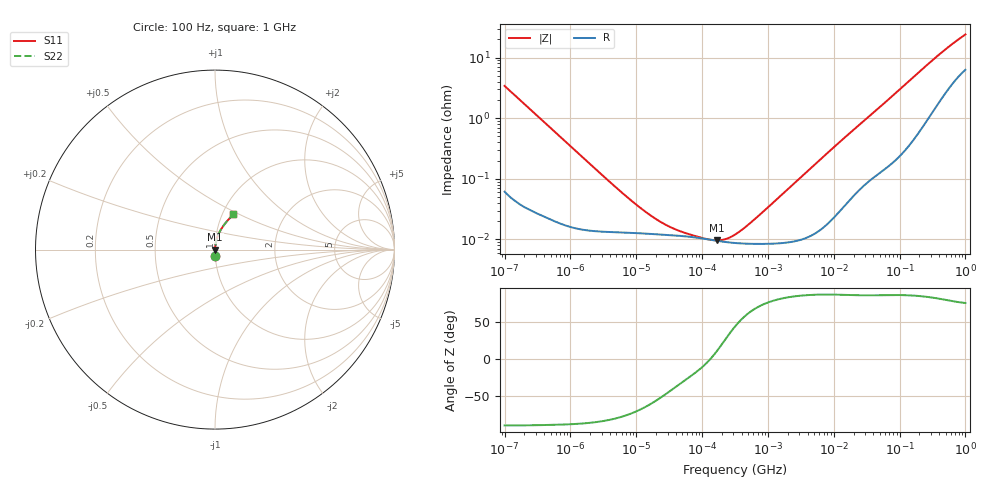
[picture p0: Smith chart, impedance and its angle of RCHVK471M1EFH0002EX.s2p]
! RCHVK471M1EFH0002EX  S-PARAMETER MODEL  (AEC-Q200 qualified)
! Model Generated by ELNA Corporation (http://www.ty-top.com)
! Version 1.0
! ELNA Control No. 240315
! Copyright (c) 2020 ELNA CO.,LTD. All Rights Reserved.
! Products Name : CONDUCTIVE POLYMER HYBRID ALUMINUM ELECTROLYTIC CAPACITORS
! Characteristics :
!  Capacitance  :  470uF  ,  Rated voltage  :  16V
!  Operating Temp. Range  :  -55 to +125 degC  ,  Endurance  :  4000hr at 125 degC
!  Dimension D  :  10mm  ,  Dimension L  :  10mm
! Frequency Range : 100Hz - 1GHz
! External Node Assignments :
!  1  o---| |---o  2
# MHz S RI R 50
!Freq[MHz].  S11 Real  S11 Imag  S21 Real  S21 Imag  S12 Real  S12 Imag  S22 Real  S22 Imag
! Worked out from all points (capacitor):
!   401 points, 100 Hz to 1 GHz, reference 50 ohm
!   read as one part in series: C = 467 uF near 108 Hz
!   lowest |Z| = 9.67 mohm at 166 kHz (marker M1)
!   series resonance near 133.9 kHz, so ESL is about 3 nH
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0.0001  0.00177 -0.034  0.9982 0.034  0.9982 0.034  0.00177 -0.034
0.000113  0.00145 -0.0302  0.9985 0.0302  0.9985 0.0302  0.00145 -0.0302
0.000309  0.000392 -0.0111  0.9996 0.0111  0.9996 0.0111  0.000392 -0.0111
0.001488  0.000151 -0.00233  0.9998 0.00233  0.9998 0.00233  0.000151 -0.00233
0.008082  0.000129 -0.000435  0.9999 0.000435  0.9999 0.000435  0.000129 -0.000435
0.013646  0.000125 -0.000261  0.9999 0.000261  0.9999 0.000261  0.000125 -0.000261
0.022131  0.000121 -0.000162  0.9999 0.000162  0.9999 0.000162  0.000121 -0.000162
0.034475  0.000117 -0.000103  0.9999 0.000103  0.9999 0.000103  0.000117 -0.000103
0.05821  0.000112 -5.7e-05  0.9999 5.7e-05  0.9999 5.7e-05  0.000112 -5.7e-05
0.115478  0.000102 -1.06e-05  0.9999 1.06e-05  0.9999 1.06e-05  0.000102 -1.06e-05
0.165959  9.53e-05 1.67e-05  0.9999 -1.67e-05  0.9999 -1.67e-05  9.53e-05 1.67e-05
0.229087  9.07e-05 4.61e-05  0.9999 -4.61e-05  0.9999 -4.61e-05  9.07e-05 4.61e-05
0.316228  8.75e-05 8.26e-05  0.9999 -8.26e-05  0.9999 -8.26e-05  8.75e-05 8.26e-05
0.436516  8.56e-05 0.000129  0.9999 -0.000129  0.9999 -0.000129  8.56e-05 0.000129
0.653131  8.46e-05 0.000207  0.9999 -0.000207  0.9999 -0.000207  8.46e-05 0.000207
4.704354  0.00012 0.00157  0.9999 -0.00157  0.9999 -0.00157  0.00012 0.00157
13.96368  0.00036 0.00456  0.9996 -0.00456  0.9996 -0.00456  0.00036 0.00456
69.9842  0.00209 0.0209  0.9979 -0.0209  0.9979 -0.0209  0.00209 0.0209
176.8072  0.00754 0.0509  0.9925 -0.0509  0.9925 -0.0509  0.00754 0.0509
380.1894  0.0272 0.1014  0.9728 -0.1014  0.9728 -0.1014  0.0272 0.1014
668.3439  0.0633 0.1541  0.9367 -0.1541  0.9367 -0.1541  0.0633 0.1541
1000  0.102 0.1961  0.898 -0.1961  0.898 -0.1961  0.102 0.1961
